ORGANIZATION_BLOCK "RACK_FLT"
TITLE = "Loss Of Rack Fault"
//Include this to prevent PLC from going to STOP due to a rack fault, i.e. a
//Profibus-DP Slave missing on the bus.
//Rack fault error handling goes here in real world applications
VERSION : 0.1


VAR_TEMP
  OB86_EV_CLASS : BYTE ;	//16#38/39 Event class 3
  OB86_FLT_ID : BYTE ;	//16#C1/C4/C5, Fault identification code
  OB86_PRIORITY : BYTE ;	//26/28 (Priority of 1 is lowest)
  OB86_OB_NUMBR : BYTE ;	//86 (Organization block 86, OB86)
  OB86_RESERVED_1 : BYTE ;	//Reserved for system
  OB86_RESERVED_2 : BYTE ;	//Reserved for system
  OB86_MDL_ADDR : WORD ;	//Depending on fault identification code
  OB86_RACKS_FLTD : ARRAY  [0 .. 31 ] OF BOOL ;	//Racks in fault
  OB86_DATE_TIME : DATE_AND_TIME ;	//Date and time OB86 started
END_VAR
BEGIN
NETWORK
TITLE =



END_ORGANIZATION_BLOCK

